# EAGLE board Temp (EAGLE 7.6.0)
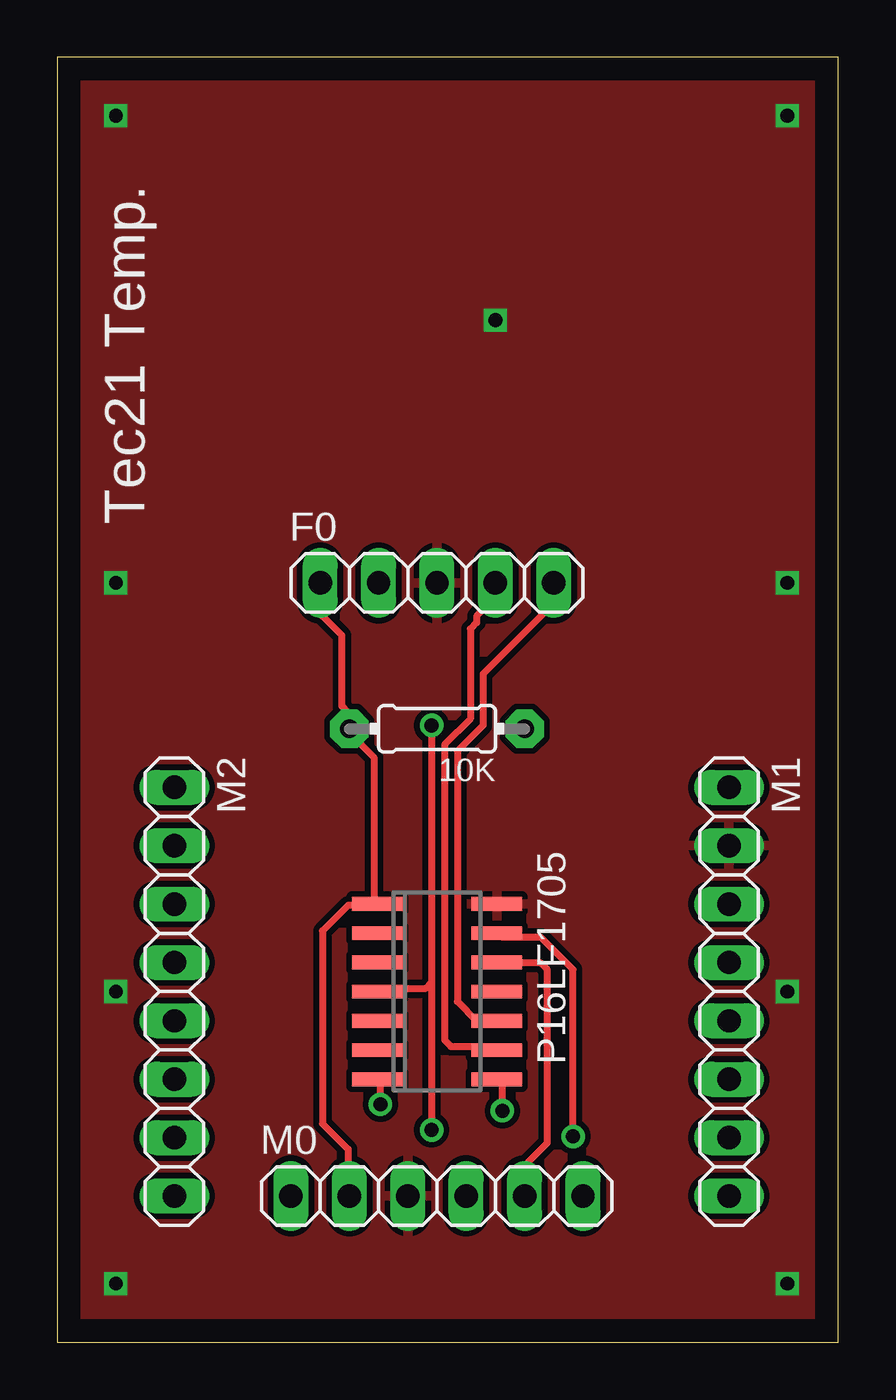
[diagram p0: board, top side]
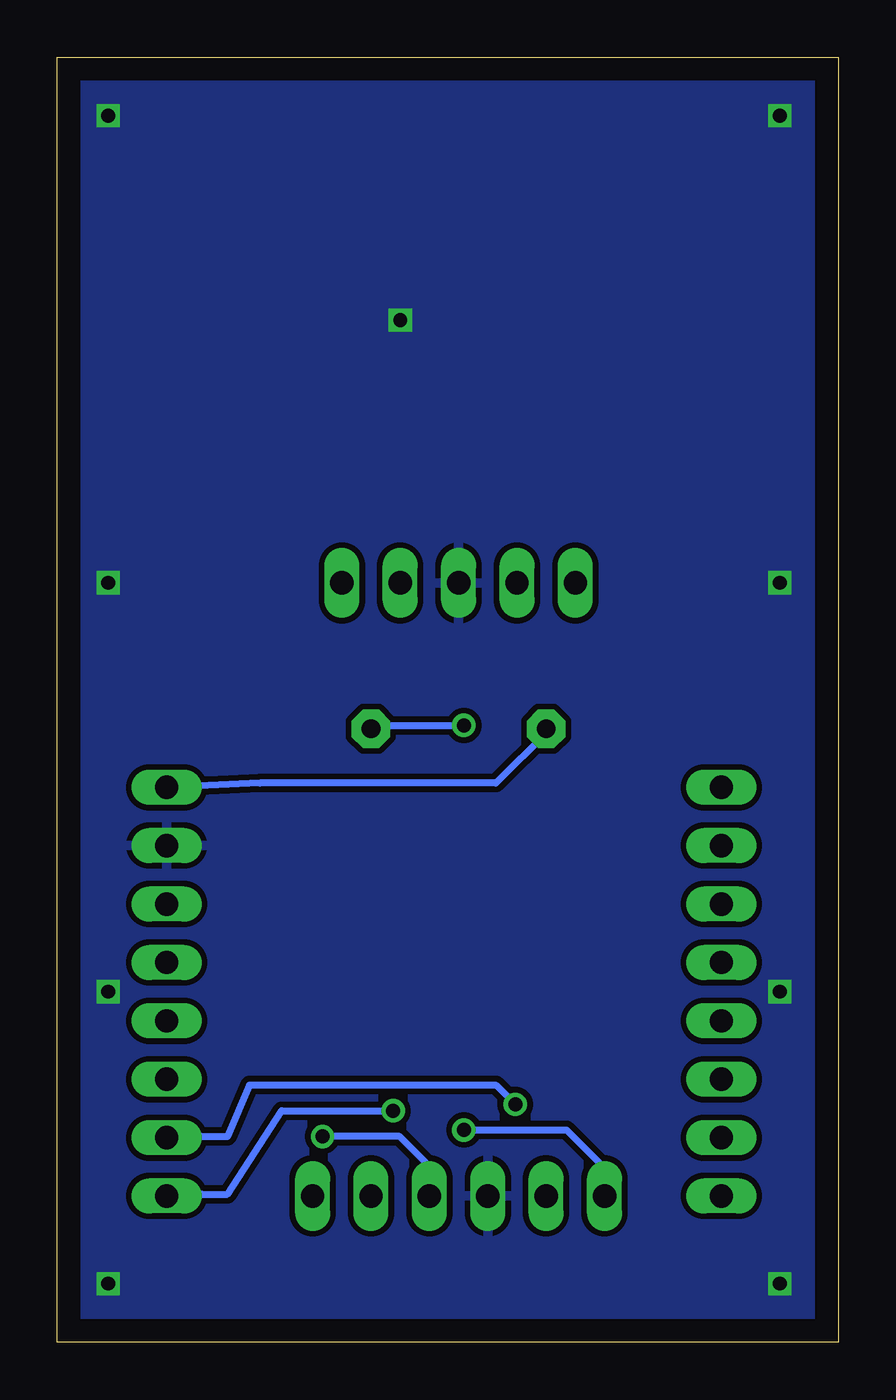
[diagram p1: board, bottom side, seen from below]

Size 33.96 x 55.87 mm. Coordinates in mm from the lower left corner, seen from the top.
Outline: 0,0 33.96,0 33.96,55.87 0,55.87 0,0
Copper layers (1*16): Top 0.035mm / dielectric 1.5mm / Bottom 0.035mm
Design rules "default": minimum track width 10mil, minimum drill 24mil, track to track 8mil, track to pad 8mil, pad to pad 8mil, via to via 8mil, smd to smd 8mil, copper to edge 40mil, drill to drill 8mil, minimum pad ring 10mil, minimum via ring 8mil, stop-mask expansion 4mil, vias tented up to drill 0mil, thermal gap 10mil
Net classes: 0 default: width 0.305 mm, drill 0.61 mm, clearance 0.254 mm

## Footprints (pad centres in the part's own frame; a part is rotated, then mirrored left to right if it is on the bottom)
0204/7 = drill 0.813 pad 1.676 octagon: 1 -3.81,0; 2 3.81,0
1X05 = drill 1.016 long: 1 -5.08,0; 2 -2.54,0; 3 0,0; 4 2.54,0; 5 5.08,0
1X06 = drill 1.016 long: 1 -6.35,0; 2 -3.81,0; 3 -1.27,0; 4 1.27,0; 5 3.81,0; 6 6.35,0
1X08 = drill 1.016 long: 1 -8.89,0; 2 -6.35,0; 3 -3.81,0; 4 -1.27,0; 5 1.27,0; 6 3.81,0; 7 6.35,0; 8 8.89,0
SO-14 = smd 0.6 x 2.2: 1 -3.81,-2.6; 2 -2.54,-2.6; 3 -1.27,-2.6; 4 0,-2.6; 5 1.27,-2.6; 6 2.54,-2.6; 7 3.81,-2.6; 8 3.81,2.6; 9 2.54,2.6; 10 1.27,2.6; 11 0,2.6; 12 -1.27,2.6; 13 -2.54,2.6; 14 -3.81,2.6

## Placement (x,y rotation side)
10K  10k  [0204/7]  16.51,26.67 180 top
F0  [1X05]  16.51,33.02 0 top
M0  [1X06]  16.51,6.35 0 top
M1  [1X08]  29.21,15.24 270 top
M2  [1X08]  5.08,15.24 270 top
P16LF1705  PIC16F676SL  [SO-14]  16.51,15.24 270 top

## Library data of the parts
10K = adafruit
F0 M0 M1 M2 = pinhead
P16LF1705 = microchip; MF: MICROCHIP; MPN: PIC16F676-I/SL; OC_FARNELL: 9760520; OC_NEWARK: 92C4557

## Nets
CCL: M1.7 P16LF1705.7
CDA: M1.8 P16LF1705.8
GND: F0.3 M0.3 M1.2 P16LF1705.14
LCL: F0.5 P16LF1705.10
LDA: F0.4 P16LF1705.9
MCLR: 10K.1 M0.1 P16LF1705.4
O3: F0.2
PGC: M0.5 P16LF1705.12
PGD: M0.4 P16LF1705.13
VDD: 10K.2 F0.1 M0.2 M1.1 P16LF1705.1

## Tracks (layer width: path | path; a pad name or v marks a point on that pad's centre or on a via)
CCL  (via drill 0.61)
  Top 0.305: v14.05,10.34 14.05,11.18 P16LF1705.7
  Bottom 0.305: v14.05,10.34 14.88,11.18 25.6,11.18 26.57,8.94 27.69,8.94 M1.7
CDA  (via drill 0.61)
  Top 0.305: v19.35,10.06 19.35,11.18 P16LF1705.8
  Bottom 0.305: v19.35,10.06 24.21,10.06 26.57,6.43 27.69,6.43 M1.8
GND  (via drill 0.6)
  other vias: 2.54,53.34 2.54,33.02 2.54,2.54 31.75,2.54 31.75,33.02 31.75,53.34 19.05,44.45 2.54,15.24 31.75,15.24
  pour Top: -1.27,57.15 35.56,57.15 35.56,-1.27 -1.27,-1.27
  pour Bottom: -1.27,57.15 35.56,57.15 35.56,-1.27 -1.27,-1.27
LCL
  Top 0.305: P16LF1705.10 18.24,13.97 17.4,14.81 17.4,25.7 18.52,26.82 18.52,29.06 21.59,32.13 F0.5
LDA
  Top 0.305: P16LF1705.9 19.08,12.85 17.12,12.85 16.84,13.13 16.84,25.98 17.96,27.1 17.96,31.01 18.24,31.29 18.24,31.57 18.8,32.13 18.8,32.97 F0.4
MCLR  (via drill 0.61)
  Top 0.305: 16.28,15.65 16,15.37 14.05,15.37 P16LF1705.4 | v16.28,26.82 16.28,15.65 | 16.28,15.65 v16.28,9.22
  Bottom 0.305: v16.28,26.82 20.19,26.82 10K.1 | v16.28,9.22 11.81,9.22 10.41,7.82 10.41,6.43 M0.1
PGC
  Top 0.305: P16LF1705.12 19.35,16.48 21.03,16.48 21.31,16.2 21.31,8.66 20.47,7.82 20.47,6.43 M0.5
PGD  (via drill 0.61)
  Top 0.305: v22.43,8.94 22.43,16.2 21.03,17.6 19.35,17.6 P16LF1705.13
  Bottom 0.305: v22.43,8.94 19.08,8.94 17.96,7.82 17.96,6.43 M0.4
VDD
  Top 0.305: F0.1 11.53,32.97 11.53,31.57 12.37,30.73 12.37,27.66 12.65,27.38 12.65,26.82 10K.2 12.93,26.54 12.93,26.26 13.77,25.43 13.77,19.28 P16LF1705.1 13.77,19 12.65,19 11.53,17.88 11.53,9.5 12.65,8.38 12.65,6.43 M0.2
  Bottom 0.305: M1.1 25.15,24.31 14.88,24.31 12.65,26.54 10K.2

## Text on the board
tPlace: Tec21 Temp.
